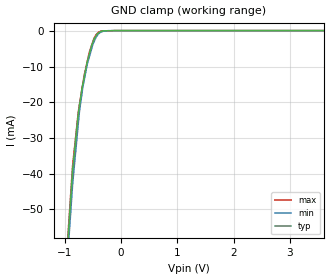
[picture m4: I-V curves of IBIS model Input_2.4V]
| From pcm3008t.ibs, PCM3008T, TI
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[Model] Input_2.4V
Model_type Input
Vinl  = 720.000mV
Vinh  = 1.68000V
C_comp  1.57000pF 1.57000pF 1.57000pF
[Model Spec]
Vinh  1.6800V  1.4700V  1.8900V
Vinl  0.7200V  0.6300V  0.8100V
| variable   typ   min   max
[Voltage Range]   2.40000V  2.10000V  2.70000V
[POWER Clamp Reference]  2.40000V  2.10000V  2.70000V
[GND Clamp Reference]   0.00000V  0.00000V  0.00000V
[Temperature Range]   25   85   -25
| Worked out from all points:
|   GND clamp passes 1 mA (typ) near -0.43 V on its own axis
[GND Clamp]
-2.4V     -403.9mA   -398.4mA   -402.3mA
-861.2mV  -39.09mA   -43.06mA   -37.84mA
-760mV    -23.24mA   -25.98mA   -22.75mA
-739.7mV  -21.04mA   -22.56mA   -20.75mA
-679.1mV  -14.99mA   -15.79mA   -14.77mA
-658.8mV  -13.33mA   -14.11mA   -12.77mA
-603mV    -8.765mA   -9.509mA   -8.771mA
-562.2mV  -6.374mA   -7.203mA   -5.847mA
-481.6mV  -2.353mA   -3.092mA   -2.118mA
-400.7mV  -568.8uA   -831.3uA   -392uA
-230mV    21.11uA    55.28uA    17.93uA
4.8V      82.58uA    62.55uA    72.72uA
[POWER Clamp]
| Voltage   I(typ)   I(min)   I(max)
-2.7V     0A         0A         0A
-2.6V     0A         0A         0A
-2.5V     0A         0A         0A
5.4V      0A         0A         0A
